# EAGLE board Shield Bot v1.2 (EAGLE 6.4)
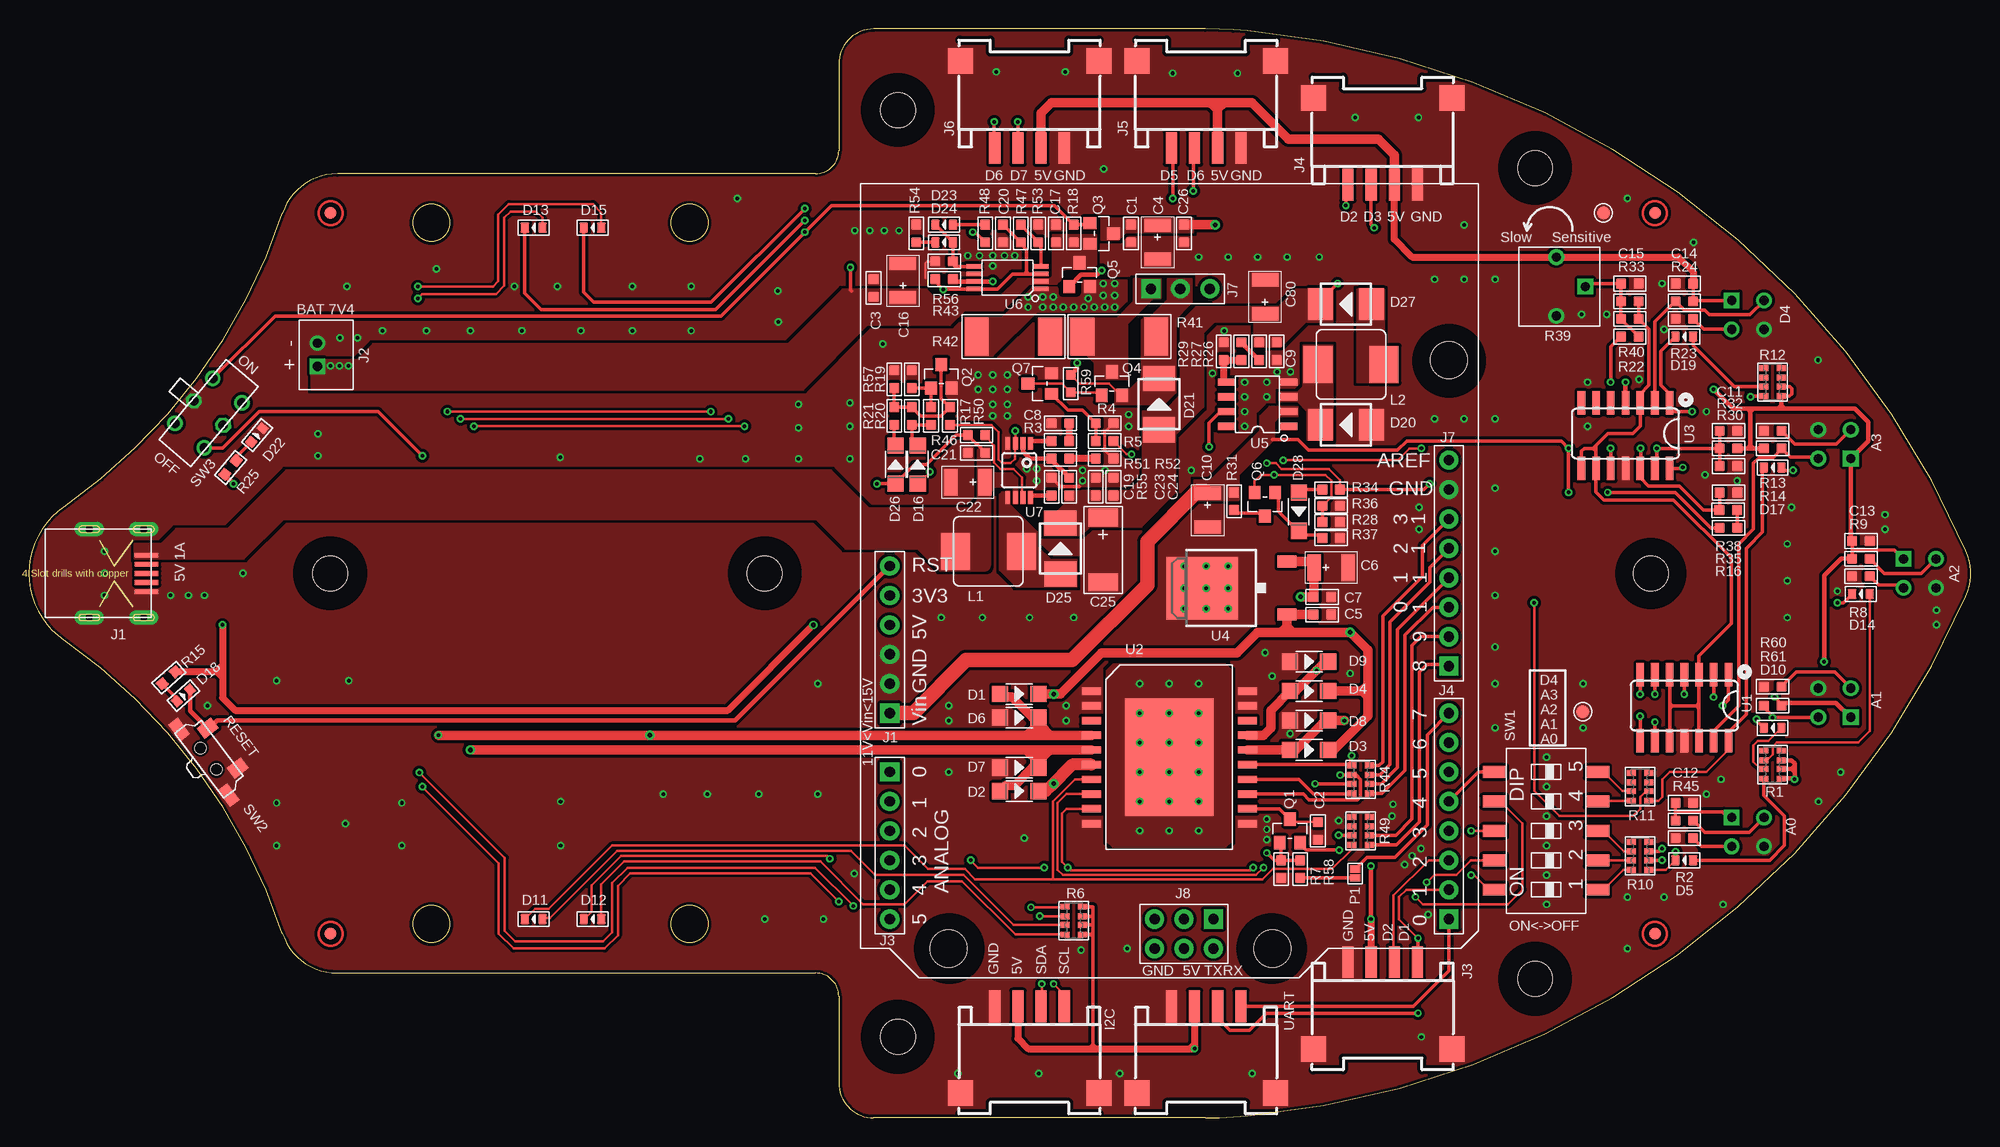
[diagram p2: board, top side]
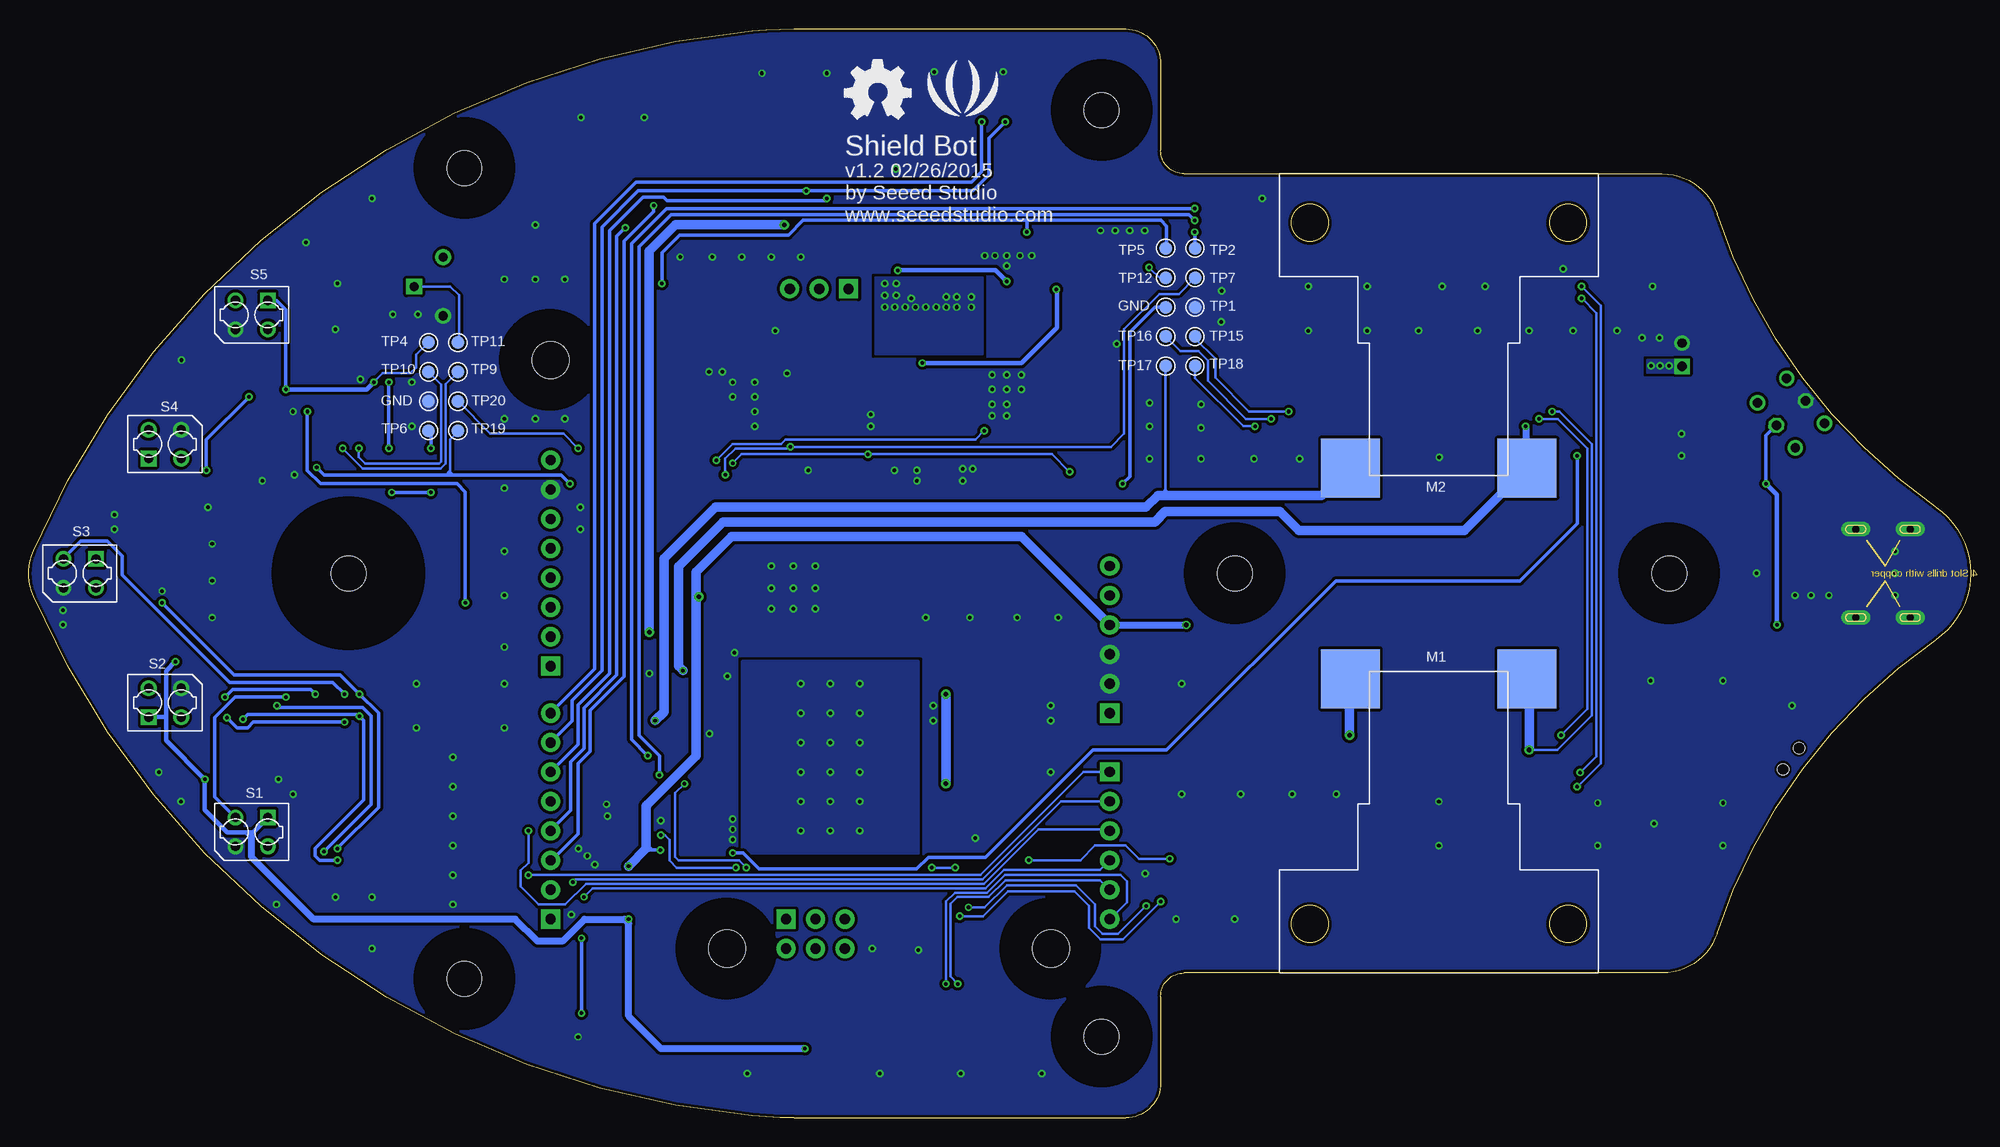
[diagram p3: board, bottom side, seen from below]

Size 167.58 x 94 mm. Coordinates in mm from the lower left corner, seen from the top.
Outline: 67.9,81.5 26.62,81.5 arc72 21.88,78.07 arc-37 3,52.74 arc110 3,41.26 arc-37 21.88,15.93 arc72 26.62,12.5 67.9,12.5 arc-90 69.9,10.5 69.9,3 arc90 72.9,0 101.53,0 arc5 105.15,0.16 arc61 167.17,45.01 arc47 167.17,48.99 arc61 105.15,93.84 arc5 101.53,94 72.9,94 arc90 69.9,91 69.9,83.5 arc-90 67.9,81.5
Outline: circle at 34.73,16.73 radius 1.6
Outline: circle at 57.02,16.73 radius 1.6
Outline: circle at 57.02,77.27 radius 1.6
Outline: circle at 34.73,77.27 radius 1.6
Copper layers (1*16): Top 0.035mm / dielectric 1.5mm / Bottom 0.035mm
Design rules "SeeedStudio_rule_no_angle_090911 *": minimum track width 6mil, minimum drill 12mil, track to track 6mil, track to pad 6mil, pad to pad 6mil, via to via 6mil, smd to smd 0mil, copper to edge 10mil, drill to drill 10mil, minimum pad ring 10mil, minimum via ring 6mil, stop-mask expansion 2mil, vias tented up to drill 25mil, thermal gap 10mil
Net classes: 0 default: width 0.203 mm, drill 0.305 mm, clearance 0.127 mm
Holes 3 mm at 26,47 63.5,47 75,87 130,82 130,12 75,7 140,47
tRestrict: area 137.2,44.2 to 142.8,49.8; area 60.7,44.2 to 66.3,49.8; area 72.2,4.2 to 77.8,9.8; area 127.2,9.2 to 132.8,14.8; area 72.2,84.2 to 77.8,89.8; area 127.2,79.2 to 132.8,84.8; area 23.2,44.2 to 28.8,49.8; area 76.8,12 to 82.1,17.3; area 104.6,12 to 109.9,17.3; area 119.8,62.6 to 125.4,68.2
bRestrict: area 133.6,40.6 to 146.3,53.3; area 22,43 to 30,51; area 71,83 to 79,91; area 126,78 to 134,86; area 59.5,43 to 67.5,51; area 71,3 to 79,11; area 126,8 to 134,16; area 75.4,10.6 to 83.4,18.6; area 103.4,10.6 to 111.4,18.6; area 118.6,61.4 to 126.6,69.4

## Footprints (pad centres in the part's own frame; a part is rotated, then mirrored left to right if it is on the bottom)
C0603 = smd 0.889 x 0.889: 1 -0.762,0; 2 0.762,0
AVX-B = smd 1.143 x 2.286: + -1.46,0; - 1.46,0
AVX-C = smd 1.524 x 2.54: + -2.794,0; - 2.794,0
SOD123 = smd 1.397 x 1.397: + -1.651,0; - 1.651,0
LED-0603 = smd 0.762 x 0.889: + -0.762,0; - 0.762,0
SMB = smd 2.159 x 2.743: + -2.21,0; - 2.21,0
4P-SMD-2.0-90D = smd 0.965 x 2.74: 1 -3,-0.1; 2 -1,-0.1; 3 1,-0.1; 4 3,-0.1 | smd 2.159 x 2.184: SS1 -5.974,7.4; SS2 5.974,7.4
MINI-SMD-5P = smd 2.032 x 0.406: 1 0.381,-1.575; 2 0.381,-0.787; 3 0.381,0; 4 0.381,0.787; 5 0.381,1.575 | drill 0.635 pad 1.27 long: GND@1 0.635,3.81; GND@2 5.334,3.81; GND@3 5.334,-3.81; GND@4 0.635,-3.81
JST-2.0 = drill 0.8 pad 1.3 square: 1 -1,0.75 | drill 0.8 pad 1.3: 2 1,0.75
3P-2.54 = drill 0.889 pad 1.651 square: 1 0,2.54 | drill 0.889 pad 1.651: 2 0,0; 3 0,-2.54
L0630 = smd 2.5 x 3.2: 1 -2.85,0; 2 2.85,0
2P-SMD-27X26 = smd 5.08 x 5.08: 1 7.62,25.4; 2 -7.62,25.4
2P-SMD-1.78X1.27 = smd 0.889 x 0.61: 1 0,0.381; 2 0,-0.381
ROUND-MARK-1.0 = smd 1.016 x 1.016: P$1 0,0
SOT23 = smd 1.016 x 1.143: 1 -0.889,-1.016; 2 0.889,-1.016; 3 0,1.016
1206-8-3.3X2.4 = smd 0.508 x 0.762: 1 -1.206,-0.762; 2 -0.381,-0.762; 3 0.381,-0.762; 4 1.206,-0.762; 5 1.206,0.762; 6 0.381,0.762; 7 -0.381,0.762; 8 -1.206,0.762
R0603 = smd 0.889 x 0.889: 1 -0.762,0; 2 0.762,0
3P-SQUA-7X6.8 = drill 0.8 pad 1.35: 1 -2.54,-0.25; 2 2.54,-0.25 | drill 0.8 pad 1.35 square: 3 0,2.25
R2512 = smd 2.032 x 3.302: 1 -3.175,0; 2 3.175,0
4P-6.4X4.9X6.5H = drill 0.8 pad 1.35 square: 1 -1.4,-1.25 | drill 0.8 pad 1.35: 2 -1.4,1.25; 3 1.4,-1.25; 4 1.4,1.25
10P-SMD-14.2X6.8 = smd 1.016 x 2.032: 1 -5.08,-4.445; 2 -2.54,-4.445; 3 0,-4.445; 4 2.54,-4.445; 5 5.08,-4.445; 6 5.08,4.445; 7 2.54,4.445; 8 0,4.445; 9 -2.54,4.445; 10 -5.08,4.445
4P-SMD-7X3.5X3.5H = smd 1.143 x 1.524: 1 -2.159,1.524; 2 2.159,1.524 | smd 1.778 x 1.016: S1 -3.556,-0.508; S2 3.556,-0.508 | hole 0.95: -1.15,0; 1.15,0
6P-2CH-2.54-9.0X3.6-90D = drill 0.813 pad 1.27: CH1A -2.54,-1.65; CH1B 2.54,-1.65; CH2A -2.54,1.65; CH2B 2.54,1.65 | drill 0.813 pad 1.27 octagon: COM1 0,-1.65; COM2 0,1.65
TP_4545 = smd 1.143 x 1.143: T 0,0
SO014 = smd 0.66 x 2.032: 1 -3.175,-2.68; 2 -1.905,-2.68; 3 -0.635,-2.68; 4 0.635,-2.68; 5 1.905,-2.68; 6 3.175,-2.68; 7 4.445,-2.68; 8 4.445,2.997; 9 3.175,2.997; 10 1.905,2.997; 11 0.635,2.997; 12 -0.635,2.997; 13 -1.905,2.997; 14 -3.175,2.997
POWERSO20 = smd 1.651 x 0.635: P$1 -6.731,5.715; P$2 -6.731,4.445; P$3 -6.731,3.175; P$4 -6.731,1.905; P$5 -6.731,0.635; P$6 -6.731,-0.635; P$7 -6.731,-1.905; P$8 -6.731,-3.175; P$9 -6.731,-4.445; P$10 -6.731,-5.715; P$11 6.731,-5.715; P$12 6.731,-4.445; P$13 6.731,-3.175; P$14 6.731,-1.905; P$15 6.731,-0.635; P$16 6.731,0.635; P$17 6.731,1.905; P$18 6.731,3.175; P$19 6.731,4.445; P$20 6.731,5.715 | smd 7.62 x 10.16: THERMALS 0,0
TO252 = smd 1.016 x 1.651: 1 -2.286,-4.826; 2 2.286,-4.826 | smd 5.4 x 6.2: 3 0,2.5
SOP8 = smd 0.635 x 1.524: 1 -1.905,-2.667; 2 -0.635,-2.667; 3 0.635,-2.667; 4 1.905,-2.667; 5 1.905,2.667; 6 0.635,2.667; 7 -0.635,2.667; 8 -1.905,2.667
TSSOP8 = smd 0.4 x 1.27: 1 -0.975,-2.9; 2 -0.325,-2.9; 3 0.325,-2.9; 4 0.975,-2.9; 5 0.975,2.9; 6 0.325,2.9; 7 -0.325,2.9; 8 -0.975,2.9
MSOP8 = smd 0.4 x 1.1: 1 -0.975,-2.35; 2 -0.325,-2.35; 3 0.325,-2.35; 4 0.975,-2.35; 5 0.975,2.35; 6 0.325,2.35; 7 -0.325,2.35; 8 -0.975,2.35
ARDUINO = drill 0.889 pad 1.651 square: 1 63.5,50.8; 9 41.656,50.8; 17 50.8,2.54; 23 45.72,2.54; 36 63.5,30.48 | drill 0.889 pad 1.651: 2 60.96,50.8; 3 58.42,50.8; 4 55.88,50.8; 5 53.34,50.8; 6 50.8,50.8; 7 48.26,50.8; 8 45.72,50.8; 10 39.116,50.8; 11 36.576,50.8; 12 34.036,50.8; 13 31.496,50.8; 14 28.956,50.8; 15 26.416,50.8; 16 23.876,50.8; 18 53.34,2.54; 19 55.88,2.54; 20 58.42,2.54; 21 60.96,2.54; 22 63.5,2.54; 24 43.18,2.54; 25 40.64,2.54; 26 38.1,2.54; 27 35.56,2.54; 28 33.02,2.54; 31 66.04,30.48; 32 66.04,27.94; 33 66.04,25.4; 34 63.5,25.4; 35 63.5,27.94 | hole 3.2: 15.24,50.8; 66.04,35.56; 66.04,7.62

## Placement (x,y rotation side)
C1  100nF  [C0603]  95.12,76.34 90 top
C2  100nF  [C0603]  111.25,24.77 270 top
C3  100nF  [C0603]  72.9,71.64 90 top
C4  22uF_16V  [AVX-B]  97.41,75.57 270 top
C5  100nF  [C0603]  111.63,43.44 0 top
C6  22uF_16V  [AVX-B]  112.39,47.51 0 top
C7  100nF  [C0603]  111.63,44.97 0 top
C8  10nF  [C0603]  89.03,59.95 180 top
C9  100nF  [C0603]  107.69,66.18 270 top
C10  22uF_16V  [AVX-B]  101.73,52.46 270 top
C11  100nF  [C0603]  146.68,59.32 0 top
C12  100nF  [C0603]  142.87,27.19 0 top
C13  100nF  [C0603]  158.11,49.79 0 top
C14  100nF  [C0603]  142.87,72.02 180 top
C15  10nF  [C0603]  138.17,72.02 180 top
C16  22uF_16V  [AVX-B]  75.44,72.27 90 top
C17  100nF  [C0603]  88.64,76.34 270 top
C19  100nF  [C0603]  88.26,54.49 90 top
C20  100nF  [C0603]  84.07,76.34 90 top
C21  100nF  [C0603]  81.79,57.41 0 top
C22  22uF_16V  [AVX-B]  81.02,54.87 180 top
C23  100nF  [C0603]  92.07,54.49 270 top
C24  100nF  [C0603]  93.6,54.49 90 top
C25  100uF_16V  [AVX-C]  92.71,49.03 270 top
C26  100nF  [C0603]  99.69,76.34 90 top
C80  22uF_16V  [AVX-B]  106.68,70.88 90 top
D1  LL4148  [SOD123]  85.47,36.59 0 top
D2  LL4148  [SOD123]  85.47,28.2 0 top
D3  LL4148  [SOD123]  110.49,31.76 0 top
D4  LL4148  [SOD123]  110.49,36.84 0 top
D5  blue  [LED-0603]  142.87,22.23 180 top
D6  LL4148  [SOD123]  85.47,34.55 0 top
D7  LL4148  [SOD123]  85.47,30.24 0 top
D8  LL4148  [SOD123]  110.49,34.3 0 top
D9  LL4148  [SOD123]  110.49,39.38 0 top
D10  blue  [LED-0603]  150.49,33.66 180 top
D11  red  [LED-0603]  43.56,17.15 180 top
D12  green  [LED-0603]  48.64,17.15 180 top
D13  red  [LED-0603]  43.56,76.84 180 top
D14  blue  [LED-0603]  158.11,45.22 180 top
D15  green  [LED-0603]  48.64,76.84 180 top
D16  LL4148  [SOD123]  76.71,56.4 90 top
D17  blue  [LED-0603]  150.49,56.14 180 top
D18  red  [LED-0603]  13.33,36.46 41.5 top
D19  blue  [LED-0603]  142.87,67.45 180 top
D20  SS54B  [SMB]  113.66,59.83 180 top
D21  SS54B  [SMB]  97.53,61.6 90 top
D22  green  [LED-0603]  19.68,58.94 50 top
D23  green  [LED-0603]  78.99,77.1 180 top
D24  red  [LED-0603]  78.99,75.57 180 top
D25  SS54B  [SMB]  89.03,49.16 90 top
D26  LL4148  [SOD123]  74.8,56.4 90 top
D27  SS54B  [SMB]  113.66,70.24 180 top
D28  LL4148  [SOD123]  109.6,52.33 270 top
I2C  [4P-SMD-2.0-90D]  86.36,9.53 180 top
J1  [MINI-SMD-5P]  10.54,47 180 top
J2  [JST-2.0]  25.65,65.87 90 top
J3  [4P-SMD-2.0-90D]  116.84,13.34 180 top
J4  [4P-SMD-2.0-90D]  116.84,80.65 0 top
J5  [4P-SMD-2.0-90D]  101.6,83.83 0 top
J6  [4P-SMD-2.0-90D]  86.36,83.83 0 top
J7  DNP  [3P-2.54]  99.38,71.57 90 top
L1  10uH  [L0630]  82.8,48.9 180 top
L2  10uH  [L0630]  114.11,65.03 0 top
M1  [2P-SMD-27X26]  45.9,12.5 0 bottom
M2  [2P-SMD-27X26]  45.9,81.5 180 bottom
P1  [2P-SMD-1.78X1.27]  114.47,21.09 0 top
P2  [ROUND-MARK-1.0]  26.03,78.11 0 top
P3  [ROUND-MARK-1.0]  140.33,15.88 0 top
P4  [ROUND-MARK-1.0]  26.03,15.88 0 top
P5  [ROUND-MARK-1.0]  140.33,78.11 0 top
Q1  NCE3407A  [SOT23]  108.84,24.77 0 top
Q2  S9013  [SOT23]  78.74,64.02 0 top
Q3  NCE3407A  [SOT23]  92.58,76.34 270 top
Q4  NCE3407A  [SOT23]  93.47,63.38 0 top
Q5  NCE3407A  [SOT23]  90.68,72.78 0 top
Q6  S9013  [SOT23]  106.68,52.97 180 top
Q7  S9013  [SOT23]  87.25,63.38 90 top
R1  4.7k  [1206-8-3.3X2.4]  150.49,30.49 90 top
R2  1k  [R0603]  142.87,24.14 0 top
R3  4.7k  [R0603]  89.03,58.43 0 top
R4  100k  [R0603]  92.84,59.95 180 top
R5  4.7k  [R0603]  92.84,58.43 0 top
R6  1k  [1206-8-3.3X2.4]  90.17,17.03 270 top
R7  100k  [R0603]  108.08,21.47 90 top
R8  1k  [R0603]  158.11,46.75 0 top
R9  47k  [R0603]  158.11,48.27 180 top
R10  1k  [1206-8-3.3X2.4]  139.06,22.62 90 top
R11  1k  [1206-8-3.3X2.4]  139.06,28.58 90 top
R12  4.7k  [1206-8-3.3X2.4]  150.49,63.51 90 top
R13  1k  [R0603]  150.49,59.32 0 top
R14  47k  [R0603]  150.49,57.79 180 top
R15  4.7k  [R0603]  12.06,37.98 41.5 top
R16  10k  [R0603]  146.68,50.94 0 top
R17  4.7k  [R0603]  77.85,60.59 270 top
R18  100k  [R0603]  90.17,76.34 90 top
R19  100k  [R0603]  76.2,63.76 90 top
R20  DNP  [R0603]  76.2,60.59 90 top
R21  4.7k  [R0603]  74.67,60.59 90 top
R22  10k  [R0603]  138.17,67.45 180 top
R23  1k  [R0603]  142.87,68.97 0 top
R24  47k  [R0603]  142.87,70.49 0 top
R25  1k  [R0603]  17.4,56.14 230 top
R26  10k  [R0603]  106.17,66.18 270 top
R27  20k_1%  [R0603]  104.65,66.18 90 top
R28  4.7k  [R0603]  112.39,51.44 0 top
R29  4.7k  [R0603]  103.12,66.18 90 top
R30  47k  [R0603]  146.68,56.27 0 top
R31  0R  [R0603]  104.01,53.22 270 top
R32  47k  [R0603]  146.68,57.79 0 top
R33  DNP  [R0603]  138.17,70.49 0 top
R34  1k  [R0603]  112.39,54.24 0 top
R35  20k_1%  [R0603]  146.67,52.46 0 top
R36  100k  [R0603]  112.39,52.84 0 top
R37  100k  [R0603]  112.39,50.05 0 top
R38  10k  [R0603]  146.68,53.98 0 top
R39  100k  [3P-SQUA-7X6.8]  132.08,71.76 270 top
R40  DNP  [R0603]  138.17,68.97 0 top
R41  1w_0.15R 1%  [R2512]  94.11,67.45 180 top
R42  1w_0.15R 1%  [R2512]  84.96,67.45 180 top
R43  1k  [R0603]  78.99,72.4 0 top
R44  1k  [1206-8-3.3X2.4]  114.93,29.22 90 top
R45  47k  [R0603]  142.87,25.66 180 top
R46  1k  [R0603]  81.79,58.94 180 top
R47  4.7k  [R0603]  85.6,76.34 270 top
R48  10k  [R0603]  82.55,76.34 270 top
R49  1k  [1206-8-3.3X2.4]  114.93,24.77 90 top
R50  10k  [R0603]  79.5,60.59 270 top
R51  20k_1%  [R0603]  89.03,56.91 180 top
R52  0R  [R0603]  92.84,56.91 180 top
R53  4.7k  [R0603]  87.12,76.34 270 top
R54  4.7k  [R0603]  76.58,76.34 270 top
R55  120k %1  [R0603]  89.79,54.49 90 top
R56  1k  [R0603]  78.99,73.92 0 top
R57  DNP  [R0603]  74.67,63.76 270 top
R58  10k  [R0603]  109.73,21.47 90 top
R59  100k  [R0603]  89.91,63.38 270 top
R60  1k  [R0603]  150.49,37.22 0 top
R61  47k  [R0603]  150.49,35.57 0 top
S1  RPR-220  [4P-6.4X4.9X6.5H]  148.37,24.68 180 bottom
S2  RPR-220  [4P-6.4X4.9X6.5H]  155.84,35.84 0 bottom
S3  RPR-220  [4P-6.4X4.9X6.5H]  163.19,47 180 bottom
S4  RPR-220  [4P-6.4X4.9X6.5H]  155.84,58.16 0 bottom
S5  RPR-220  [4P-6.4X4.9X6.5H]  148.37,69.32 180 bottom
SW1  DM-05  [10P-SMD-14.2X6.8]  130.94,24.77 90 top
SW2  BUTTON-4P-REINFORCE'TS-1188E'  [4P-SMD-7X3.5X3.5H]  15.49,31 307 top
SW3  [6P-2CH-2.54-9.0X3.6-90D]  15.49,60.84 230 top
TP1  [TP_4545]  69.47,69.99 270 bottom
TP2  [TP_4545]  66.93,75.07 270 bottom
TP3  [TP_4545]  133.09,61.86 0 bottom
TP4  [TP_4545]  133.09,66.94 270 bottom
TP5  [TP_4545]  69.47,75.07 270 bottom
TP6  [TP_4545]  133.09,59.32 270 bottom
TP7  [TP_4545]  66.93,72.53 270 bottom
TP8  [TP_4545]  66.93,69.99 0 bottom
TP9  [TP_4545]  130.55,64.4 270 bottom
TP10  [TP_4545]  133.09,64.4 270 bottom
TP11  [TP_4545]  130.55,66.94 270 bottom
TP12  [TP_4545]  69.47,72.53 270 bottom
TP13  [TP_4545]  134.11,35.06 0 top
TP14  [TP_4545]  135.89,78.11 0 top
TP15  [TP_4545]  66.93,67.45 0 bottom
TP16  [TP_4545]  69.47,67.45 0 bottom
TP17  [TP_4545]  69.47,64.91 0 bottom
TP18  [TP_4545]  66.93,64.91 0 bottom
TP19  [TP_4545]  130.55,59.32 0 bottom
TP20  [TP_4545]  130.55,61.86 0 bottom
U1  LMV324-SO014  [SO014]  143.51,35.57 180 top
U2  L298P  [POWERSO20]  98.42,31.12 0 top
U3  LMV324-SO014  [SO014]  138.43,59.06 180 top
U4  CJ78M05  [TO252]  103.76,45.73 90 top
U5  TD1410  [SOP8]  106.04,61.6 90 top
U6  BQ2057WTS  [TSSOP8]  84.45,72.53 90 top
U7  ISL97516  [MSOP8]  85.47,55.89 180 top
U8  [ARDUINO]  71.75,80.65 270 top
U$1  [LOGO_SILK]  86.99,88.15 0 bottom
U$2  [OSHW_FILLX200_NOTEXT]  97.15,86.24 0 bottom
UART  [4P-SMD-2.0-90D]  101.6,9.53 180 top

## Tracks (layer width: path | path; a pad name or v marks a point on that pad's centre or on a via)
5V  (via drill 0.3, 0.3 pad 0.64, 0.38 pad 0.81, 0.41 pad 0.64)
  Top 0.203: 142.24,27.06 C12.1
  Top 0.305: v142.87,36.59 U1.4 | R6.8 91.82,18.23 91.82,18.04 | 91.82,18.04 91.82,17.54 | 91.82,17.54 91.82,17.41 | 91.82,17.41 91.69,17.41 | 91.69,17.41 R6.7 | R6.6 91.69,16.65 | 91.69,16.65 91.82,16.65 | 91.82,16.65 91.82,16.77 | 91.82,16.77 91.82,17.28 | 91.82,17.28 91.82,17.41 | 91.82,15.82 91.82,16.01 | 91.82,16.01 91.82,16.52 | 91.82,16.52 91.82,16.65 | R6.5 91.64,15.82 | 91.64,15.82 91.82,15.82 | 91.82,15.82 91.82,15.63 | 91.82,15.63 91.82,6.36 | 91.82,6.36 91.82,5.98 | R12.2 151.96,63.13 152.14,62.95 152.14,62.49 151.95,62.3 R12.1 | C14.1 R24.2 | R24.2 | R24.2 143.71,70.57 S5.1 | v113.07,23.12 110.23,23.12 109.73,23.63 Q1.2 | S3.1 161.01,49.03 157.35,49.03 | 157.35,49.03 | 157.35,49.03 C13.1 | R9.2 157.35,49.03 | R61.2 151.26,35.74 v150.66,36.33 | S1.1 146.67,25.93 146.18,26.43 142.11,26.43 | 142.11,26.43 C12.1 | C12.1 | 142.11,26.43 R45.2 | 91.82,6.36 92.07,6.11 | 91.82,6.36 91.57,6.11 | 91.82,18.04 91.69,18.17 | 91.69,17.41 91.82,17.28 | 91.69,17.41 91.82,17.54 | 91.69,16.65 91.82,16.77 | 91.69,16.65 91.82,16.52 | 91.64,15.82 91.64,15.81 91.82,15.63 | 91.64,15.82 91.64,15.83 91.82,16.01
  Top 0.406: U3.4 v137.79,63.51 | R32.2 148.33,57.79 | 148.33,57.79 148.72,57.79 | 148.72,57.79 148.84,57.79 | 148.84,57.79 R14.2 | S2.1 157.19,34.59 155.95,35.82 151.51,35.82 R61.2 | v154.94,39.38 154.94,46.8 156.4,48.27 R9.2 | 12.7,38.62 12.7,38.55 R15.2 | R1.3 152.11,30.87 152.4,30.59 152.4,30.36 | 152.4,30.36 152.4,30.11 | 152.4,30.11 152.4,29.85 | 152.4,29.85 152.4,29.47 | 152.4,29.47 v152.4,29.22 | v152.4,29.22 | R1.1 152.21,29.28 | 152.21,29.28 152.34,29.28 v152.4,29.22 | R1.2 152.14,30.11 | 152.14,30.11 152.4,30.11 | 152.4,30.11 | 152.14,30.11 | 152.14,30.11 152.4,30.36 | 152.14,30.11 152.4,29.85 | 152.21,29.28 152.4,29.47 | v115.82,21.73 v115.82,17.15 | v145.41,62.87 | 148.33,61.22 147.06,61.22 v145.41,62.87 | 148.33,61.22 148.59,60.97 | 148.59,60.97 148.84,61.22 | 148.84,61.22 151,61.22 | 151,61.22 151.26,61.22 | 151.26,61.22 151.51,61.22 | 151.51,61.22 157.61,61.22 158.75,60.08 158.75,58.43 157.24,56.92 S4.1 157.24,49.79 C13.1 | R12.1 151.26,61.48 | 151.26,61.48 151.26,61.22 | 148.59,60.97 148.59,58.05 | 148.59,58.05 148.59,57.92 148.72,57.79 | 151,61.22 151.26,61.48 | 148.84,57.79 148.59,58.05 | 148.33,57.79 148.59,58.05 | 148.33,61.22 148.84,61.22 | 151.26,61.48 151.51,61.22 | R25.2 16.91,55.49 v17.65,54.75
  Top 0.61: I2C.3 85.36,6.85 86.23,5.98 91.82,5.98 100.2,5.98 | 100.2,5.98 v100.6,5.98 UART.3 100.58,9.62 | v115.82,17.15 115.82,13.46 J3.3 | C14.1 143.64,73.03 142.37,74.3 R39.1 119.38,74.3 117.84,75.84 J4.3 | C14.1 | 100.2,5.98 100.58,6.36 | v67.69,42.55 60.32,35.19 17.78,35.19 16.7,36.27 16.7,38.62 | v16.7,42.55 16.7,38.62 | 12.7,38.55 16.19,38.55 | 16.19,38.55 16.64,38.55 16.7,38.62 | 16.19,38.55 16.64,39 16.64,38.11 16.19,38.55 | 16.19,38.55
  Top 0.813: J6.3 87.36,86.73 88.26,87.64 102.61,87.64 | 102.61,87.64 103.12,87.64 | 103.12,87.64 105.54,87.64 108.71,84.46 116.46,84.46 117.84,83.08 J4.3 | J5.3 102.6,87.02 | 102.6,87.12 102.6,87.62 102.61,87.64 | 102.6,87.02 102.11,87.51 | 102.6,87.02 102.6,87.12 | 102.6,87.12 103.12,87.64 | v109.77,44.97 C7.1 110.91,45.01 110.91,47.53 | U4.2 110.53,48.02 110.91,47.63 110.91,47.53 | 110.91,47.53 C6.+
  Bottom 0.203: 148.33,24.52 148.33,24.65 | 114.17,27.06 114.3,26.93 | v137.79,63.51 137.79,63.55 137.07,64.27 134.66,64.27 134.15,64.78 134.15,65.88 TP4.T
  Bottom 0.305: v150.66,36.33 150.62,36.33 149.99,36.97 143.25,36.97 v142.87,36.59 | v145.41,62.87 145.41,69.77 146.22,70.57 S5.1 | SW3.COM2 17.65,58.89 v17.65,54.75 | v113.07,23.12 113.79,23.12 | 113.79,23.12 114.17,23.12 arc90 114.3,23.25 | 113.79,23.12 114.04,23.38
  Bottom 0.406: S1.1 146.97,25.89 148.21,24.65 148.33,24.65 148.84,24.65 | 148.84,24.65 150.45,24.65 152.4,26.59 v152.4,29.22 155.74,32.56 155.74,34.68 | 155.74,34.68 155.74,38.58 v154.94,39.38 | 155.74,34.68 155.83,34.59 S2.1 | v145.41,62.87 138.43,62.87 v137.79,63.51 | 148.84,24.65 148.46,24.27 | v16.7,42.55 16.7,53.8 v17.65,54.75
  Bottom 0.61: v100.6,5.98 113.03,5.98 115.82,8.77 115.82,16.77 | U8.26 v67.69,42.55 | 148.33,24.52 148.33,22.49 143,17.15 125.6,17.15 123.7,15.25 121.54,15.25 119.63,17.15 116.2,17.15 | 148.33,24.52 | 115.82,16.77 v115.82,17.15 116.2,17.15 | 115.82,16.77 116.2,17.15
  Bottom 0.813: U8.26 81.91,50.17 106.93,50.17 109.98,47.13 109.98,45.18 v109.77,44.97 109.98,44.75 | U8.26 | 114.3,26.93 114.3,23.25 v115.82,21.73 | 114.17,27.06 109.98,31.25 109.98,44.75 | 109.98,44.75 109.98,45.69
A0  (via drill 0.3 pad 0.64)
  Top 0.203: v124.46,20.96 124.71,20.96 125.73,19.95 126.24,19.95 SW1.10
  Bottom 0.203: U8.17 76.58,29.85 85.47,20.96 v124.46,20.96
A1  (via drill 0.3 pad 0.64)
  Top 0.203: 125.86,22.11 126.11,22.11 | 126.11,22.11 126.36,22.11 SW1.9 | v120.65,20.33 121.28,20.96 123.19,20.96 124.46,22.23 125.98,22.23 126.11,22.11
  Bottom 0.203: U8.18 78.52,27.31 85.26,20.58 120.39,20.58 v120.65,20.33
A2  (via drill 0.3 pad 0.64)
  Top 0.203: v124.46,24.77 SW1.8 | SW1.8
  Bottom 0.203: U8.19 74.42,24.9 80.43,24.9 85.13,20.2 119.51,20.2 121.28,18.42 123.59,18.42 125.13,19.97 125.13,21.35 124.46,22.02 v124.46,24.77
A3  (via drill 0.3)
  Top 0.203: v119.67,19.06 120.31,18.42 127.63,18.42 128.9,19.69 128.9,25.41 126.87,27.44 126.62,27.44 SW1.7
  Bottom 0.203: v119.67,19.06 118.91,19.82 85,19.82 83.41,21.41 75.12,21.41 U8.20
A4/SDA  (via drill 0.3)
  Top 0.203: v87.41,11.57 87.41,10.42 87.36,10.37 I2C.2
  Bottom 0.203: U8.21 75.12,20.52 83.29,20.52 84.75,19.06 87.45,19.06 88.05,18.46 88.05,12.2 v87.41,11.57
A5/SCL  (via drill 0.3 pad 0.64)
  Top 0.203: v88.43,11.57 89.45,10.55 89.36,10.46 I2C.1
  Bottom 0.203: U8.22 72.83,18.62 72.83,20.42 73.37,20.96 83.35,20.96 84.87,19.44 87.67,19.44 88.43,18.68 v88.43,11.57
BOOST_EN  (via drill 0.3 pad 0.64)
  Top 0.203: R50.2 83.06,59.83 83.69,59.19 83.69,56.81 83.98,56.52 84.73,56.52 85.09,56.88 85.09,58.18 U7.3 85.13,58.26 v85.13,59.32 | v108.24,56.78 118.15,56.78 119.16,57.79 v120.18,57.79
  Bottom 0.203: v85.13,59.32 85.89,58.56 102.27,58.56 102.65,58.18 106.85,58.18 v108.24,56.78 | v120.18,57.79 121.45,59.06 127.76,59.06 TP20.T 130.55,61.56
D0/RX
  Top 0.305: UART.1 119.48,9.63 122.55,12.71 U8.1
D1/TX  (via drill 0.3)
  Top 0.203: 119.67,14.49 119.67,13.61 J3.1 | U8.2 118.87,19.69 118.24,19.06 118.24,17.15 v119.89,15.5
  Top 0.305: UART.2 102.6,8.62 103.66,7.56 105.34,7.56 106.81,9.03 v119.89,9.03 | v119.89,15.5 119.89,13.49 J3.1
  Bottom 0.305: v119.89,9.03 v119.89,15.5
D2  (via drill 0.3 pad 0.64)
  Top 0.203: U8.3 120.81,22.23 117.77,19.19 117.77,13.52 J3.2
  Top 0.305: v113.66,78.75 113.66,80.38 J4.1
  Bottom 0.305: v113.66,78.75 | U8.3 122.47,22.23 120.18,24.52 120.18,30.62 119.16,31.63 119.16,35.15 116.2,38.11 116.2,75.7 113.66,78.24 v113.66,78.75
D3  (via drill 0.3 pad 0.64)
  Top 0.305: J4.2 115.84,77.12 v116.12,76.84
  Bottom 0.305: U8.4 122.55,24.81 120.82,26.55 120.82,30.74 119.67,31.89 119.67,35.4 116.84,38.24 116.84,76.12 v116.12,76.84
D4
  Top 0.305: SW1.6 125.09,29.85 U8.5
D5  (via drill 0.3 pad 0.64)
  Top 0.305: 98.55,83.68 J5.1 98.72,83.61 v98.72,79.38
  Bottom 0.305: U8.6 120.18,32.23 120.18,35.66 117.47,38.36 117.47,76.57 114.56,79.48 112.79,79.48 112.49,79.19 98.91,79.19 v98.72,79.38
D6  (via drill 0.3 pad 0.64)
  Top 0.305: 100.58,83.71 J5.2 100.5,83.73 v100.5,80.02 | 83.31,83.76 J6.1 83.31,83.78 v83.31,85.99
  Bottom 0.305: U8.7 120.69,34.26 120.69,36.04 118.11,38.62 118.11,76.89 114.98,80.02 v100.5,80.02 86.1,80.02 84.71,81.42 84.71,84.59 v83.31,85.99
D7  (via drill 0.3 pad 0.64)
  Top 0.305: 85.34,83.71 J6.2 | 85.26,83.63 85.34,83.71 | 85.34,83.71 v85.34,85.99 | U8.8 120.69,33.07 120.69,25.28 117.89,22.49 115.48,22.49 P1.1
  Bottom 0.305: U8.8 118.74,38.74 118.74,77.21 115.17,80.78 86.23,80.78 85.34,81.67 v85.34,85.99 | v85.34,85.99
ENA  (via drill 0.3 pad 0.64)
  Top 0.203: 91.01,27.95 89.53,27.95 88.77,27.19 88.77,21.42 89.23,20.96 105.92,20.96 v106.55,21.6
  Top 0.305: U2.P$8 91.01,27.95 | R49.7 v113.03,24.39
  Bottom 0.203: v113.03,24.39 112.69,24.39 112.31,24.01 112.31,22.23 111.67,21.6 v106.55,21.6
ENB
  Top 0.305: U2.P$14 109.6,29.22 110.87,27.95 114.11,27.95 R44.8
FAST_CHAR  (via drill 0.3 pad 0.64)
  Top 0.203: R34.2 113.16,55.04 112.18,56.02 108.12,56.02 107.61,56.52 v106.85,56.52 | D16.+ 76.75,54.75 v77.76,55.76 | v95.16,57.29 94.74,57.29 R5.2
  Top 0.305: v142.75,56.14 142.75,56.07 U3.14 | v120.9,54.75 120.39,54.24 R34.2
  Bottom 0.203: v106.85,56.52 106.08,57.29 v95.16,57.29 79.29,57.29 v77.76,55.76 | 130.72,59.32 TP19.T 130.55,59.23 131.23,58.56 131.23,55.82 | 131.23,55.8 131.23,55.51 | 131.23,55.82 131.26,55.82 131.57,55.51 | 131.23,55.82 131.23,55.8 | 131.23,55.8 130.94,55.51
  Bottom 0.305: v142.75,56.14 142.11,55.51 131.57,55.51 131.23,55.51 130.94,55.51 121.66,55.51 v120.9,54.75
GND  (via drill 0.3 pad 0.64)
  Top 0.203: 77.38,72.49 77.38,73.8 77.51,73.92 R56.1
  Top 0.254: R52.1 92.84,57.67 92.84,59.19 R4.1
  Top 0.305: C19.2 89.03,54.49 90.68,54.49
  other vias: 79.37,29.85 85.89,24.14 79.37,35.57 117.73,27.06 120.14,23.25 106.68,40.14 107.31,38.11 114.04,38.36 144.78,27.95 146.05,29.22 137.96,14.61 160.19,50.81 156.08,45.48 140.97,72.02 108.58,74.3 100.96,74.3 103.5,74.3 106.04,74.3 83.18,61.6 89.53,34.3 89.53,35.57 83.18,74.43 86.99,55 90.93,55.89 90.93,55 86.99,56.02 83.18,62.87 152.14,52.71 151.76,49.54 151.76,46.36 151.76,43.19 120.78,17.54 119.38,22.62 118.74,21.85 90.8,14.49 103.5,45.73 99.69,45.73 99.69,43.95 101.6,43.95 103.5,43.95 79.37,34.3 108.84,33.16 113.03,25.66 144.78,60.97 144.65,55.51 147.45,55 94.78,14.61 120.18,6.99 105.58,3.82 94.15,3.82 87.16,3.82 80.18,3.82 45.89,27.31 45.89,23.5 6.52,47 6.52,45.09 6.52,48.9 117.64,26.04 154.43,65.41 143.68,75.57 137.96,79.38 119.93,86.37 114.47,86.37 104.31,90.18 98.72,90.18 89.45,90.31 83.48,90.31 92.75,81.92 68.07,27.95 62.99,27.95 58.55,27.95 54.74,27.95 68.07,37.47 61.85,56.91 45.85,57.03 27.43,71.76 26.84,67.32 28.36,67.32 24.93,59.06 24.93,57.16 32.17,27.19 32.17,23.5 21.38,23.5 21.38,27.19 21.38,37.73 27.6,37.73 18.45,47 134.15,37.47 134.15,33.66 126.53,33.66 126.53,37.47 126.53,40.65 126.53,45.09 126.53,48.9 126.53,54.37 136.18,69.35 134.53,63.51 123.86,77.1 138.98,63.76 141.14,68.08 160.19,52.08 164.63,43.82 164.63,42.55 156.38,29.85 154.47,27.31 146.22,18.42 141.14,19.06 137.96,19.06 73.7,66.81 61.13,79.38 64.68,68.72 83.18,73.54 84.2,74.43 106.85,62.24 104.94,59.7 104.94,60.97 104.94,62.24 106.85,63.51 104.94,63.51 119.99,52.71 119.99,50.81 130.98,18.42 130.98,20.96 130.98,23.5 130.98,26.04 130.98,28.58 130.98,31.12 134.53,59.7 86.1,56.02 57.91,56.91 121.32,72.4 123.86,72.4 126.53,72.4 121.32,60.33 123.86,60.33 126.53,60.33 71.25,21.09 13.76,45.09 12.23,45.09 15.15,45.09 99.69,47.63 103.5,47.63 101.6,45.73 101.6,47.63 103.16,67.95 102.15,64.27 106.85,24.9 106.85,25.79 106.85,24.01 72.56,76.59 75.1,76.59 73.83,76.59 71.29,76.59 94.91,59.7 94.91,60.72 92.88,55.89 84.45,61.6 82.04,74.43 81.02,74.43 30.52,67.95 34.29,67.95 38.1,67.95 47.62,67.95 52.07,67.95 57.15,67.95 64.64,71.38 52.07,71.76 57.15,71.76 35.18,73.29 41.91,71.76 42.54,67.95 45.59,71.76 63.5,17.15 68.58,17.15 27.3,25.41 100.33,55.89 86.36,43.19 90.17,43.19 82.29,43.19 78.74,43.19 107.74,64.4 108.88,64.4 84.45,62.87 66.42,56.91 66.42,59.57 66.42,61.6 70.86,61.73 70.86,59.7 70.86,56.91 111.38,74.3 134.02,69.35 85.09,74.43 81.91,62.87 83.18,64.14 81.91,64.14 83.18,60.59 84.45,60.59 84.45,64.14 15.41,35.57
  pour Top (isolate 0.203, rank 6, no thermals): 84.07,59.95 84.66,59.95 84.66,57.16 84.07,57.16
  pour Bottom (isolate 0.254, rank 6, no thermals): -2.67,-3.17 169.67,-3.17 169.67,96.4 -2.67,96.4
  pour Top (isolate 0.254, rank 6, no thermals): -2.67,-3.17 169.67,-3.17 169.67,96.4 -2.67,96.4
  pour Top (isolate 0.254, rank 6, no thermals): 106.21,38.11 104.31,38.11 104.31,35.32 106.21,35.32
  pour Top (isolate 0.254, rank 6, no thermals): 92.62,38.24 90.72,38.24 90.72,35.44 92.62,35.44
  pour Top (isolate 0.254, rank 6, no thermals): 106.21,25.66 104.43,25.66 104.43,22.87 106.21,22.87
  pour Top (isolate 0.254, rank 6, no thermals): 92.37,25.66 90.46,25.66 90.46,22.87 92.37,22.87
GREF
  Top 0.305: 135.25,57.54 U3.9 135.25,54.03 135.94,53.35 141.94,53.35 146.94,48.35 146.94,42.68 144.14,39.89 144.14,38.5 144.27,38.38 U1.3 144.14,35.57 | 135.25,57.54 135.25,57.79 | 135.25,57.79 135.25,58.05 | U3.3 139.06,59.7 138.43,59.06 136.27,59.06 135.25,58.05 | U3.8 133.98,57.54 134.24,57.79 135,57.79 | 135,57.79 135.25,57.79 | 135,57.79 135.25,58.05 | 135,57.79 135.25,57.54 | 141.6,35.57 141.6,35.32 | 141.6,35.32 U1.10 | 144.14,35.57 U1.12 | U1.5 141.6,35.82 | 141.6,35.82 141.6,35.57 | 141.6,35.57 141.86,35.57 | 141.86,35.57 143.89,35.57 | 143.89,35.57 144.14,35.57 | 141.86,35.57 141.6,35.82 | 141.86,35.57 141.6,35.32 | 139.19,61.87 U3.3 | 143.89,35.57 144.14,35.82 144.14,35.32 143.89,35.57 | U3.3 139.06,62.49 139.83,63.26 139.83,68.08 R40.2 | U3.3 | R33.2 R40.2 | R40.2
IN1
  Top 0.203: 90.93,29.22 U2.P$7 90.3,29.22 88.39,27.31 88.39,20.71 | 88.39,20.58 88.39,20.71 | 88.52,20.58 88.39,20.58 | 88.39,20.58 88.26,20.58 | 88.26,20.58 81.66,20.58 80.77,21.47 77.6,21.47 75.56,23.5 50.33,23.5 44.87,18.04 43.69,18.04 D11.- 42.92,17.28 | 42.92,17.28 | 88.39,20.71 88.52,20.58 | 88.39,20.71 88.26,20.58 | 88.52,20.58 106.46,20.58 107.35,21.47 112.46,21.47 114.17,23.18 R49.8
IN2  (via drill 0.3, 0.3 pad 0.64)
  Top 0.203: U2.P$9 89.53,26.68 89.15,26.3 89.15,22.11 v89.66,21.6 89.91,21.35 105.41,21.35 v105.66,21.6 | v87.63,21.6 81.91,21.6 v81.28,22.23 | D12.- | D12.- 47.92,17.15 48.55,17.79 48.55,20.08 51.09,22.62 68.87,22.62 v69.13,22.36
  Top 0.305: R44.7 v111,28.84
  Bottom 0.203: v89.66,21.6 v87.63,21.6 | v81.28,22.23 76.83,22.23 75.56,23.5 72.94,23.5 71.79,22.36 v69.13,22.36 | v105.66,21.6 106.3,22.23 111.51,22.23 111.8,22.52 111.8,28.04 v111,28.84
IN3  (via drill 0.3 pad 0.64)
  Top 0.203: 105.28,28.08 U2.P$13
  Top 0.305: v113.16,29.6 R44.6 114.55,29.6 114.93,29.22 114.93,27.7 114.68,27.44 110.49,27.44 109.98,27.95 U2.P$13 105.15,28.08 | D13.- 42.8,71.19 44.22,69.77 59.26,69.77 v66.97,77.48
  Bottom 0.305: v113.16,29.6 113.16,31.25 114.93,33.03 114.93,75.2 112.14,77.99 67.48,77.99 v66.97,77.48
IN4  (via drill 0.3 pad 0.64)
  Top 0.305: U2.P$15 114.11,30.49 | 114.11,30.49 R44.5 | 114.11,30.49 114.11,31.19 v114.17,31.25 | D15.- 47.88,71.27 48.75,70.4 58.87,70.4 v66.97,78.5
  Bottom 0.305: v114.17,31.25 115.57,32.65 115.57,75.45 112.53,78.5 v66.97,78.5
LINE-FINDER-1  (via drill 0.3 pad 0.64)
  Top 0.203: R10.1 141.29,21.41 D5.-
  Top 0.305: U1.1 146.68,36.08 v146.18,35.57 | v142.11,23 D5.- | D5.-
  Bottom 0.305: v146.18,35.57 146.05,35.44 138.79,35.44 138.05,34.7 138.05,27.06 v142.11,23
LINE-FINDER-2  (via drill 0.3 pad 0.64)
  Top 0.305: U1.8 v139.06,34.68 | v149.1,34.43 149.1,34.3 D10.- | R10.2 140.71,22.23 | 140.71,22.23 v140.97,22.23 | v140.97,22.23 | v140.97,22.23 140.71,22.23 | 140.71,22.23
  Bottom 0.305: v149.1,34.43 148.72,34.81 139.19,34.81 v139.06,34.68 | v140.97,22.23 142.49,22.23 142.87,22.62 142.87,23.25 138.68,27.44 138.68,34.3 v139.06,34.68 | v139.06,34.68
LINE-FINDER-3  (via drill 0.3 pad 0.64)
  Top 0.305: U1.7 v139.06,36.59 | R10.3 140.71,23 v140.97,23.25 | D14.- 156.59,44.46 v156.08,44.46
  Bottom 0.305: v156.08,44.46 | v156.08,44.46 149.86,38.24 140.71,38.24 v139.06,36.59 | v140.97,23.25 137.41,26.81 137.41,34.93 v139.06,36.59 | v139.06,36.59
LINE-FINDER-4
  Top 0.203: R11.1 140.65,27.38 140.97,27.7 140.97,29.22 141.6,29.85 144.78,29.85 146.68,31.76 U1.14 | U1.14
  Top 0.305: 148.33,49.29 149.6,50.56 149.6,55.76 149.73,55.89 D17.- | 148.33,49.29 | 148.33,49.29 148.21,49.16 148.21,34.81 146.68,33.28 U1.14 | U1.14
LINE-FINDER-5  (via drill 0.3 pad 0.64)
  Top 0.203: v129.92,44.46 129.92,28.2 132.08,26.04 138.43,26.04 139.06,26.68 139.06,27.7 139.7,28.33 | 139.7,28.33 | 139.7,28.33 R11.2
  Top 0.305: D19.- 140.84,66.18 140.84,63.26 141.6,62.49 U3.1 141.6,60.97 v143.55,60.97
  Bottom 0.305: v143.55,60.97 143.55,55.89 142.41,54.75 130.64,54.75 129.92,54.03 v129.92,44.46
LIPO-7V4  (via drill 0.38 pad 0.81, 0.41 pad 0.81)
  Top 0.813: 87.12,27.95 D2.- | D1.- v88.43,36.59 89.03,36.59 92.58,40.14 104.27,40.14 106.04,41.92 108.46,41.92 | 115.57,36.71 115.57,34.68 112.65,31.76 D3.- | D4.- 115.06,36.84 | 115.06,36.84 115.44,36.84 115.57,36.71 | 108.46,41.92 109.09,41.92 | 109.09,41.92 v114.04,41.92 115.57,40.4 115.57,36.71 | v88.43,28.84 88.39,28.84 88.16,28.6 | C5.1 U4.1 108.58,42.43 | 108.58,42.43 108.58,42.05 108.46,41.92 | v102.4,77.1 C26.2 | 108.58,42.43 | 108.58,42.43 109.09,41.92 | 108.58,42.43 108.2,42.05 | 115.06,36.84 115.57,37.35 | 115.06,36.84 115.57,36.33
  Top 1.016: U2.P$6 90.04,30.49 88.16,28.6 87.76,28.2 D2.-
  Bottom 0.813: v114.04,41.92 114.04,74.81 111.76,77.1 v102.4,77.1 | v88.43,36.59 v88.43,28.84
  pour Top (no thermals): 100.46,77.61 92.58,77.61 92.58,75.83 94.04,75.83 94.68,76.46 100.46,76.46
LIPO-OUT-7V4  (via drill 0.3 pad 0.64)
  Top 0.305: v70.9,73.42 70.9,71.47 70.99,71.38
  Bottom 0.203: v70.9,73.42 69.89,72.4 69.59,72.4 TP12.T
  other vias: 26.03,64.91 26.8,64.91 27.56,64.91
  pour Top (no thermals): 24.38,65.41 28.32,65.41 29.72,66.81 65.53,66.81 70.23,71.51 74.95,71.51 74.95,68.46 72.39,68.46 66.8,62.87 24.38,62.87
  pour Top (rank 2, no thermals): 88.01,72.4 88.01,72.02 86.36,72.02 84.07,69.73 80.77,69.73 79.5,68.46 74.55,68.46 74.55,71.51 77.46,71.51 78.1,70.87 80.14,70.88 83.82,70.88 85.34,72.4
  pour Top (no thermals): 87.12,72.02 88.61,72.02 arc45 88.7,72.06 88.97,72.32 arc45 89.03,72.46 89.03,72.86 arc-45 89.1,73.05 89.27,73.21 arc-45 89.45,73.29 91.71,73.29 92.07,73.65 92.07,76.21 88.39,76.21 88.39,72.73 arc-45 88.34,72.61 88.18,72.45 arc-45 88.06,72.4 87.12,72.4
  pour Bottom (no thermals): 24.38,65.41 27.88,65.41 27.88,64.34 24.38,64.34
MOTOR_CTR  (via drill 0.3 pad 0.64)
  Top 0.305: R7.2 108.08,23.63 Q1.1 | R58.2 R7.2 | R7.2 107.48,22.23 v106.85,22.87 | v33.95,57.16 30.14,60.97 19.85,60.97 16.72,57.84 SW3.CH2B
  Bottom 0.305: v106.85,22.87 105.96,22.87 104.56,21.47 90.97,21.47 89.95,22.49 85,22.49 75.73,31.76 69.38,31.76 54.78,46.36 38.9,46.36 33.95,51.32 v33.95,57.16
N$1  (via drill 0.3 pad 0.64)
  Top 0.203: R6.2 v87.25,17.41 | D15.+ | v69.89,18.68 67.48,21.09 51.89,21.09 50.84,20.04 50.84,15.76 49.7,14.61 41.82,14.61 40.55,15.88 40.55,21.98 v33.95,28.58 | v33.57,71.76 40.05,71.76 40.51,72.22 40.51,77.97 41.41,78.88 48.68,78.88 49.4,78.16 D15.+
  Bottom 0.203: v87.25,17.41 85.22,17.41 83.06,19.57 77.34,19.57 76.07,18.3 76.07,16.39 75.11,15.43 73.14,15.43 v69.89,18.68 | v33.57,71.76 31.92,70.11 31.92,30.62 v33.95,28.58
N$2  (via drill 0.3 pad 0.64)
  Top 0.305: S1.3 148.48,24.65 144.65,24.65 R45.1 | v145.41,36.33 U1.2
  Bottom 0.305: S1.3 151.55,27.71 151.55,34.58 149.8,36.33 v145.41,36.33
N$3  (via drill 0.3 pad 0.64)
  Top 0.305: v140.33,34.17 U1.9 | R61.1 149.73,35.44 150.62,34.55 | v150.49,34.55 150.62,34.55 | 150.62,34.55 154.41,34.55 S2.3
  Bottom 0.305: v150.49,34.55 149.6,33.66 148.72,33.66 148.21,34.17 v140.33,34.17
N$4
  Top 0.203: D10.+ | D10.+ 150.11,32.52 149.22,32.52 148.84,32.14 148.84,30.74 149.48,30.11 R1.7 | R1.7
N$5
  Top 0.305: S1.2 144.35,23.43 R2.2
N$6
  Top 0.305: R60.2 152.53,38.49 155.84,38.49 S2.2
N$7  (via drill 0.3 pad 0.64)
  Top 0.203: v86.49,18.17 89.34,18.17 R6.1 | v71.16,18.3 67.86,21.6 51.65,21.6 50.33,20.28 50.33,16.01 49.57,15.25 41.95,15.25 41.06,16.14 41.06,22.45 v33.69,29.81 | D13.+ 44.32,77.71 43.79,78.24 41.56,78.24 41.02,77.7 41.02,71.85 40.3,71.13 33.95,71.13 v33.57,70.75
  Bottom 0.203: v86.49,18.17 85.09,18.17 83.18,20.08 77.21,20.08 75.56,18.42 75.56,16.52 74.93,15.88 73.57,15.88 v71.16,18.3 | v33.57,70.75 32.3,69.48 32.3,31.21 v33.69,29.81
N$8  (via drill 0.3 pad 0.64)
  Top 0.305: S3.3 163.34,47 160.15,47 R9.1 | U1.6 v140.33,36.59
  Bottom 0.305: v140.33,36.59 141.35,37.6 150.24,37.6 159.51,46.87 159.51,48.48 160.82,49.79 163.12,49.79 164.63,48.29 S3.3
N$9
  Top 0.203: D14.+ 158.88,33.39 157.88,32.39 150.87,32.39 150.49,32.01 150.49,31.38 149.99,30.87 R1.6 | R1.6
N$10
  Top 0.305: S3.2 161.56,45.98 159.64,45.98 R8.2 | R8.2
N$11
  Top 0.203: R6.4 85.15,15.82 80.54,20.43 77.57,20.43 75.56,18.42 72.01,18.42 68.3,22.13 51.39,22.13 49.4,20.14 D12.+
N$12
  Top 0.305: D5.+ 150.24,22.23 151.51,23.5 151.51,26.04 150.37,27.19 | 150.37,27.19 | 150.37,27.19 149.73,27.82 R1.8
N$13
  Top 0.305: 151.26,59.57 R13.2 152.4,58.18 156.01,58.18 S4.2
N$14  (via drill 0.3 pad 0.64)
  Top 0.305: R12.8 148.65,62.3 v148.59,62.24 | D17.+ 151.51,55.89 v152.27,55.89
  Bottom 0.305: v152.27,55.89 152.27,58.56 v148.59,62.24
N$15
  Top 0.203: R10.8 137.6,21.41 135.76,19.57 135.51,19.57 SW1.1
N$16
  Top 0.406: R26.2 R27.2
N$17
  Top 0.203: R10.7 SW1.2 | SW1.2 135.25,22.23 | 135.25,22.23 | 135.25,22.23 SW1.2 | SW1.2
N$18
  Top 0.305: R12.7 147.19,63.13 143.64,66.68 D19.+
N$19
  Top 0.305: S5.2 144.54,68.07 R23.2
N$20
  Top 0.305: U3.2 140.33,68.72 R24.1 142.87,69.73 144.65,69.73 145.03,69.35 148.55,69.35 S5.3
N$21
  Top 0.203: R10.6 137.67,23 135.89,24.77 SW1.3 | SW1.3
N$22
  Top 0.203: R11.8 135.44,27.38 SW1.4
N$23
  Top 0.203: R11.7 137.54,28.2 135.76,29.98 135.51,29.98 SW1.5
N$24
  Top 0.305: P1.2 R58.1
N$25
  Top 0.305: D18.+ 12.76,36.21 R15.1
N$26
  Top 0.305: R19.1 Q2.1 R17.1
N$27
  Top 0.203: U7.7 85.72,53.61 85.72,55.25 84.96,56.02 83.85,56.02 83.31,56.56 83.31,58.05 82.55,58.81 R46.1
N$28
  Top 0.203: R6.3 84.96,16.65 80.64,20.96 73.02,20.96 70.94,23.05 50.77,23.05 45,17.28 44.45,17.28 D11.+ arc-90 44.36,17.19
N$29
  pour Top (no thermals): 87.12,69 94.78,69 94.78,63.76 91.99,63.76 91.99,65.16 91.22,65.92 87.12,65.9
  pour Top (no thermals): 93.47,68.97 93.85,68.97 95.38,70.49 95.38,72.4 97.66,72.4 97.66,70.75 97.03,70.75 94.49,68.21 93.47,68.21
N$30
  Top 0.305: R35.2 147.43,50.95 R16.2
N$31
  Top 0.305: R25.1 17.89,57.05 D22.+
N$32  (via drill 0.3 pad 0.64)
  other vias: 93.72,72.02 92.71,72.02 93.72,71 93.72,69.99 92.71,71 92.84,69.99 91.06,69.99 89.28,69.99 87.5,69.99 88.39,70.88 91.95,69.99 90.17,69.99 88.39,69.99 86.23,69.99 86.23,70.88 91.44,70.75 87.5,70.88
  pour Top (rank 3, no thermals): 80.77,69.1 84.02,69.1 86.61,71.69 88.55,71.69 arc-90 88.77,71.47 88.77,69.61 86.99,69.61 83.18,65.8 80.77,65.8
  pour Top (no thermals): 87.12,69.61 87.12,71.26 88.77,71.26 88.77,71.15 arc45 88.85,70.95 88.98,70.82 arc45 89.16,70.75 90.45,70.75 arc45 90.66,70.84 90.84,71.02 arc45 90.93,71.23 90.93,72.15 91.06,72.27 94.74,72.27 94.74,70.52 93.83,69.61
  pour Bottom: 94.53,72.53 94.53,65.92 85.26,65.92 85.26,72.53
N$33
  Top 0.305: S4.3 154.32,57.03 152.02,57.03 R14.1 151.26,57.73 150.49,56.97 149.29,56.97 148.84,56.52 148.84,50.81 147.57,49.54 147.57,35.57 145.41,33.41 U1.13 | U1.13
N$34
  Top 0.305: R21.1 74.67,58.18 D26.-
N$35  (via drill 0.3 pad 0.64)
  Top 0.305: 79.81,72.2 79.81,72.34 R43.2
  Top 0.406: 79.81,72.2 U6.7 83.18,72.2 v83.18,72.21 | v92.58,73.16 92.2,72.78 90.8,72.78 Q5.1
  Bottom 0.406: v92.58,73.16 84.14,73.16 v83.18,72.21
N$36
  Top 0.305: D24.- R54.2
N$37
  Top 0.305: R53.2 | R53.2 R47.1 | U6.4 87.35,75.34 R53.2
N$38
  Top 0.305: D23.- D24.+ 79.75,75.32 79.82,75.26 | U6.5 79.92,73.5 79.75,73.67 R56.2 79.75,75.19 79.82,75.26 | 79.82,75.26 79.88,75.32
N$39
  Top 0.305: R48.1 D23.+
N$40
  Top 0.305: Q6.1 107.82,53.73 107.82,52.33 109.47,50.68 D28.- 109.98,50.3 111.38,50.3 R37.1
N$41
  Top 0.406: U7.8 86.64,53.73 C19.1
N$42
  Top 0.406: R55.2 88.26,56.78 R51.2 86.39,56.91 85.8,57.5 U7.2
N$43
  pour Top (no thermals): 90.42,45.86 85.24,45.86 83.82,47.28 83.82,53.81 84,53.98 84.58,53.98 84.58,52.99 86.99,50.58 86.99,49.34 88.19,48.14 90.42,48.14
N$44
  Top 0.406: R3.1 86.63,58.43 U7.1
N$45
  Top 0.61: R3.2 C8.1
N$46
  Top 0.305: R57.2 R21.2 R20.2 76.96,60.59 78.74,60.59 R50.1 | R50.1 | Q2.3 78.74,62.11 R50.1 | 79.37,61.35 R50.1 | R50.1
N$47  (via drill 0.3 pad 0.64)
  Top 0.305: R38.1 | v139.1,57.79 139.1,56.11 U3.12 139.06,55.22 139.1,55.22 139.76,54.56 142.43,54.56 144.52,52.46 R35.1 145.92,52.48 R38.1
  Bottom 0.203: 133.09,64.23 TP10.T 131.99,63.3 131.99,56.65 132.15,56.49 138.56,56.49 139.1,57.03 v139.1,57.79
N$48
  Top 0.305: D16.- 76.2,58.56 R20.1 R17.2
N$49  (via drill 0.3 pad 0.64)
  Top 0.305: SW3.CH1A 21.24,69.22 59.73,69.22 v66.97,76.46 69.25,78.75 88.52,78.75 R18.2 91.44,77.1 Q3.1
  Bottom 0.305: v66.97,76.46 66.93,76.42 TP2.T
N$50  (via drill 0.3 pad 0.64)
  Top 0.305: C11.1 R32.1 | R30.1 R32.1 | R32.1 v140.5,57.79 140.5,56.23 U3.13
  Bottom 0.203: v140.5,57.79 138.77,56.07 132.03,56.07 131.61,56.48 131.61,63.34 TP9.T | 130.59,64.4 TP9.T | 130.55,64.25 TP9.T
  Bottom 0.305: 130.55,64.36 TP9.T
N$51
  Top 0.61: R52.2 R51.1
N$54
  Top 0.305: Q6.3 106.68,52.21 104.01,52.21 R31.2
N$55
  pour Top (no thermals): 107.95,62.62 107.95,61.86 109.47,61.86 110.36,60.97 110.36,58.56 112.52,58.56 112.52,66.68 109.98,66.68 109.98,63.13 109.47,62.62
N$56
  Top 0.203: C2.1 109.09,25.54 Q1.3
  Top 0.305: U2.P$12 107.95,26.68 Q1.3
N$57
  Top 0.61: R27.1 R29.1 103.12,63.51 U5.5
N$58  (via drill 0.3 pad 0.64)
  Top 0.305: R22.2 136.52,66.56 v136.52,63.51 | v136.52,57.79 U3.10 | U3.10
  Bottom 0.305: v136.52,63.51 v136.52,57.79
N$59
  Top 0.305: R39.3 134.58,72.02 C15.2 R33.1 | R33.1 | R22.1 R40.1 | R33.1 R40.1 | R40.1
  Bottom 0.203: R39.3 131.23,71.76 130.47,71 130.47,67.03 TP11.T
N$61
  Top 0.305: R44.4 116.52,30.43 116.84,30.74 116.84,43.32 120.27,46.75 120.27,49.41 U8.14
N$62
  Top 0.305: R44.3 116.58,29.6 117.47,30.49 117.47,42.81 120.9,46.24 120.9,47.51 U8.13
N$63
  Top 0.305: U8.12 118.11,42.17 118.11,30.24 116.71,28.84 R44.2
N$64
  Top 0.305: R44.1 116.78,28.01 118.74,29.98 118.74,41.67 121.16,44.08 U8.11
N$65
  Top 0.305: U8.10 120.12,41.54 119.38,40.8 119.38,25.79 117.98,24.39 R49.2
N$66
  Top 0.305: U8.9 122.43,39.13 120.65,39.13 120.01,38.49 120.01,25.54 118.05,23.57 R49.1
N$70  (via drill 0.3 pad 0.64)
  Top 0.203: R36.1 112.39,53.6 112.39,55 111.89,55.51 v107.48,55.51 106.34,55.51 105.79,54.96 Q6.2 | U5.7 102.84,60.97
  Top 0.305: R28.1 R36.1 | 102.84,60.97 101.85,59.98 v101.85,57.92
  Bottom 0.203: v107.48,55.51 107.48,56.91 106.59,57.79 101.96,57.79 101.85,57.9 v101.85,57.92 | 101.7,57.79 101.83,57.92 v101.85,57.92 | TP7.T 68.32,71.13 70.02,71.13 73.06,68.08 73.06,59.06 74.21,57.92 v101.85,57.92
N$71
  pour Top (no thermals): 114.68,71.51 114.68,63.51 116.97,63.51 116.97,71.51
N$72
  Top 0.203: Q7.3 89.15,63.38 R59.2 92.33,62.62 Q4.1
N$73
  Top 0.305: R5.1 R4.2 90.93,61.1 89.66,61.1 Q7.1
N$74
  Top 0.305: R34.1 109.85,54.24 D28.+
OUT1  (via drill 0.3 pad 0.64, 0.41 pad 0.81)
  Top 0.203: v37.25,60.33 v60.36,60.33
  Top 0.813: 86.1,33.03 v53.59,33.03 v35.34,33.03 | 86.1,33.03 87.25,33.03 | 87.25,33.03 88.14,33.03 | 88.14,33.03 U2.P$4 | 87.25,33.03 87.12,33.16 D6.- 86.61,34.55 84.83,36.33 84.07,36.33 D1.+ | 88.14,33.03 87.25,33.92 | 86.1,33.03 86.99,33.92
  Bottom 0.203: v60.36,60.33 62.52,60.33 65.82,63.64 65.82,65.36 66.64,66.18 68.2,66.18 TP16.T | v37.25,60.33 35.6,60.33 33.06,57.79 33.06,35.32 v35.34,33.03
  Bottom 0.813: v53.59,33.03 53.59,37.83 M1.2
OUT2  (via drill 0.3 pad 0.64, 0.41 pad 0.81)
  Top 0.203: v36.11,60.97 v58.84,60.97
  Top 0.813: U2.P$5 86.99,31.76 | 86.99,31.76 86.1,31.76 | 86.1,31.76 v38.1,31.76 | 87.12,30.84 D7.- 86.61,30.24 85.09,28.71 84.33,28.71 D2.+ | 87.12,30.84 87.12,31.63 86.99,31.76 | 87.12,30.84 87.03,30.84 86.1,31.76 | 87.12,30.84 87.21,30.84 88.01,31.63
  Bottom 0.203: 38.1,31.89 38.1,31.85 38.01,31.76 35.64,31.76 32.68,34.72 32.68,58.15 35.5,60.97 v36.11,60.97 | v58.84,60.97 62.27,60.97 65.19,63.89 65.19,65.54 66.93,67.28 TP15.T 66.62,67.45
  Bottom 0.813: v38.1,31.76 38.1,31.89 38.1,37.72 M1.1
OUT3  (via drill 0.3 pad 0.64)
  Top 0.813: U2.P$16 D3.+ 109.35,31.76 111.76,34.17 112.01,34.17 D8.- v113.54,34.3
  Bottom 0.203: TP17.T 69.47,54.24 | 69.47,54.24 69.47,54.02 69.76,53.73 | 69.47,54.24 69.72,53.98 | 69.47,54.24 | 69.47,54.24 69.21,53.98
  Bottom 0.813: 53.34,56.27 53.35,56.27 M2.1 | 53.56,56.14 M2.1 | v113.54,34.3 112.77,35.06 112.77,48.27 108.33,52.71 71.16,52.71 70.14,53.73 69.76,53.73 56.05,53.73 53.68,56.1 M2.1
OUT4  (via drill 0.3 pad 0.64)
  Top 0.203: v38.39,59.7 v61.76,59.7
  Top 0.813: U2.P$17 106.55,33.03 107.19,33.66 107.19,35.19 D4.+ 109.35,36.84 v111.12,38.62 111.76,39.25 112.01,39.25 D9.-
  Bottom 0.203: v61.76,59.7 62.78,59.7 66.93,63.85 TP18.T
  Bottom 0.61: 38.41,56.28 38.28,56.28 M2.2 38.39,56.1 | v38.39,59.7 38.39,56.1 | 38.39,55.64 38.39,56.1
  Bottom 0.813: 38.73,55.89 38.48,56.14 38.32,56.14 M2.2 | 38.35,56.03 M2.2 | v111.12,38.62 111.5,39 111.5,47.61 107.67,51.44 70.4,51.44 69.51,52.33 59.6,52.33 57.95,50.68 43.7,50.68 M2.2 | 38.61,55.76 38.48,55.76 38.1,56.14 38.23,56.14 M2.2 | 38.44,56.1 M2.2
PAD  (via drill 0.3 pad 0.64)
  other vias: 95.88,37.47 98.42,37.47 100.96,37.47 95.88,34.93 95.88,32.39 95.88,29.85 95.88,27.31 95.88,24.77 98.42,24.77 100.96,24.77 98.42,27.31 100.96,27.31 98.42,29.85 100.96,29.85 98.42,32.39 100.96,32.39 98.42,34.93 100.96,34.93
  pour Top (isolate 0.254, no thermals): 103.75,38.62 103.75,23.89 103.24,23.38 93.59,23.38 93.08,23.89 93.08,38.62 93.59,39.13 103.24,39.13
  pour Bottom (isolate 0.254, no thermals): 90.79,39.38 106.03,39.38 106.03,22.87 90.79,22.87
RES
  Top 0.406: U8.28 60.96,34.3 16.25,34.3 15.62,33.66 15.62,33.79 | 15.18,33.86 SW2.1 15.56,33.79 15.62,33.79 | 15.18,33.86 13.9,35.15 D18.- | 15.75,33.79 15.62,33.79 | 15.37,33.92 15.24,33.92 15.18,33.86
USB_CHARGE  (via drill 0.3 pad 0.64)
  Top 0.305: v73.19,54.75 D26.+ 76.45,56.4 77.47,56.4 80.01,58.94 R46.2 C21.2
  Top 0.406: C21.2 82.55,57.54
  Bottom 0.305: v73.19,54.75 72.56,55.38 72.56,67.83 70.4,69.99 TP1.T
  pour Top (no thermals): 9.14,49.54 9.14,48.27 18.54,48.27 21.97,51.7 67.94,51.7 70.48,49.16 76.71,49.16 78.61,47.25 82.42,47.25 arc90 82.93,47.76 82.93,52.59 72.51,52.59 69.22,55.88 22.22,55.88 17.14,50.81 12.7,50.81 11.43,49.54
  pour Top (no thermals): 80.01,47.25 82.42,47.25 arc90 82.93,47.76 82.93,57.79 82.04,57.79 81.91,57.67 81.91,53.35 80.01,51.44
  pour Top (no thermals): 85.01,53.1 85.27,53.1 85.27,55.22 84.85,55.64 83.44,55.64 83.06,56.02 82.17,56.02 82.17,53.98 82.93,53.98 83.44,54.49 84.79,54.49 85.01,54.27
VCC-8V8  (via drill 0.3 pad 0.64)
  Top 0.203: 93.98,62.87 93.98,62.62 | R59.1 90.68,63.38 93.22,63.38 94.23,62.37
  Top 0.305: U6.3 86.1,72.85 | 86.1,72.85 85.92,72.85 | 85.92,72.85 84.91,72.85 83.61,71.55 U6.8 78.95,71.55 v78.91,71.51 78.23,72.19 R43.1 78.23,72.31 | R47.2 | R47.2 C20.2 | R47.2 85.6,75.45 86.1,74.94 86.1,73.03 | 86.1,73.03 86.1,72.85 | 86.1,73.03 86.23,72.91 | 85.92,72.85 86.1,73.03
  Top 0.406: v90.46,65.16 90.46,64.69 R59.1
  Bottom 0.406: v90.46,65.16 81.91,65.16 78.87,68.21 78.87,71.47 v78.91,71.51
  pour Top (no thermals): 98.97,69.1 98.97,62.62 97.95,61.6 93.77,61.6 93.77,62.87 95.03,62.87 96.05,63.89 96.05,68.88 96.27,69.1
  pour Top (no thermals): 98.3,72.4 100.33,72.4 100.33,70.37 98.8,68.84 98.8,68.08 96.26,68.08 96.26,69.1 96.75,69.1 98.3,70.65
VCC-9V  (via drill 0.3 pad 0.64)
  Top 0.305: R48.2 81.66,76.46 v81.45,76.46 | D27.- 111.45,70.53 v112.94,72.02
  Bottom 0.305: v112.94,72.02 112.94,74.69 111.42,76.21 102.02,76.21 100.75,77.48 81.45,77.48 | 81.45,77.48 69.89,77.48 69.38,76.97 69.38,75.15 TP5.T | v81.45,76.46 81.45,77.48
  pour Top (no thermals): 87.63,50.3 90.8,50.3 91.57,51.06 94.23,51.06 94.23,54.11 89.41,54.11 89.41,52.97 88.77,52.33 87.63,52.33
  pour Top (no thermals): 91.95,54.11 94.97,54.11 96.14,55.28 96.14,60.46 98.93,60.46 98.93,53.96 96.04,51.06 91.95,51.06
  pour Top (no thermals): 105.54,69.99 107.82,69.99 109.35,71.51 112.52,71.51 112.52,68.72 110.23,68.72 108.08,66.56 105.79,66.56 105.79,68.59 105.54,68.84
  pour Top (no thermals): 96.14,58.94 98.91,58.94 101.34,61.38 101.34,67.73 102.34,68.72 106.3,68.72 106.3,69.99 100.74,69.99 99.44,68.69 99.44,62.42 97.99,60.97 96.14,60.97
VIN  (via drill 0.3 pad 0.64)
  Top 0.305: v136.27,53.98 142.11,53.98 145.16,50.94 R16.1 | v132.88,53.98 v132.88,57.79 132.25,58.43 118.91,58.43 118.13,57.64 110.42,57.64 109.51,58.56 107.31,58.56
  Top 1.27: U8.23 76.33,34.93 80.9,39.51 90.03,39.51 96.52,45.99 96.52,49.77 100.86,54.11 101.54,54.11 C10.+
  Bottom 0.305: v136.27,53.98 v132.88,53.98 | 133.13,59.28 TP6.T 132.88,59.1 v132.88,57.79
  pour Top (no thermals): 100.58,55 104.39,55 104.39,53.35 100.58,53.35
  pour Top (no thermals): 104.39,53.6 104.39,55.51 107.44,58.56 107.44,60.08 107.95,60.59 109.47,60.59 109.47,61.35 107.06,61.35 106.3,60.59 106.3,59.32 101.98,55 101.98,53.6 102.12,53.61 102.11,53.6

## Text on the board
tPlace: D6 | D7 | 5V | GND | D5 | D6 | 5V | GND | D2 | D3 | 5V | GND | Slow | Sensitive | BAT 7V4 | D4 | - | ON | + | J7 | A3 | OFF | 5V 1A | A2 | D4 | A3 | J4 | A2 | A1 | RESET | A1 | A0 | J1 | 11V<Vin<15V | A0 | J8 | ON<->OFF | J3 | GND | 5V | D2 | D1 | GND | 5V | TX | RX | GND | 5V | SDA | SCL
bPlace: Shield Bot | v1.2 02/26/2015 | by Seeed Studio | www.seeedstudio.com | GND | GND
